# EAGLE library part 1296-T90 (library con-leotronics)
1.27mm SINGLE ROW FEMALE SOCKET Source: http://www.leotronics.co.uk/Conexcon/Data%20Sheets/sec.%20A/1296ing.pdf
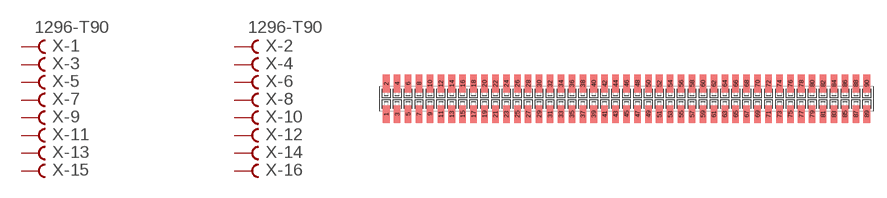
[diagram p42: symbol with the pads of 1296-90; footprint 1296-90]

Designator prefix X; gates -1=FVAL -2=FVAL -3=F -4=F -5=F -6=F -7=F -8=F -9=F -10=F -11=F -12=F -13=F -14=F -15=F -16=F -17=F -18=F -19=F -20=F -21=F -22=F -23=F -24=F -25=F -26=F -27=F -28=F -29=F -30=F -31=F -32=F -33=F -34=F -35=F -36=F -37=F -38=F -39=F -40=F -41=F -42=F -43=F -44=F -45=F -46=F -47=F -48=F -49=F -50=F -51=F -52=F -53=F -54=F -55=F -56=F -57=F -58=F -59=F -60=F -61=F -62=F -63=F -64=F -65=F -66=F -67=F -68=F -69=F -70=F -71=F -72=F -73=F -74=F -75=F -76=F -77=F -78=F -79=F -80=F -81=F -82=F -83=F -84=F -85=F -86=F -87=F -88=F -89=F -90=F

## 1296-T90 (OC_FARNELL: unknown; OC_NEWARK: unknown)  [1296-90]
1  -1:B  pas
2  -2:B  pas
3  -3:B  pas
4  -4:B  pas
5  -5:B  pas
6  -6:B  pas
7  -7:B  pas
8  -8:B  pas
9  -9:B  pas
10  -10:B  pas
11  -11:B  pas
12  -12:B  pas
13  -13:B  pas
14  -14:B  pas
15  -15:B  pas
16  -16:B  pas
17  -17:B  pas
18  -18:B  pas
19  -19:B  pas
20  -20:B  pas
21  -21:B  pas
22  -22:B  pas
23  -23:B  pas
24  -24:B  pas
25  -25:B  pas
26  -26:B  pas
27  -27:B  pas
28  -28:B  pas
29  -29:B  pas
30  -30:B  pas
31  -31:B  pas
32  -32:B  pas
33  -33:B  pas
34  -34:B  pas
35  -35:B  pas
36  -36:B  pas
37  -37:B  pas
38  -38:B  pas
39  -39:B  pas
40  -40:B  pas
41  -41:B  pas
42  -42:B  pas
43  -43:B  pas
44  -44:B  pas
45  -45:B  pas
46  -46:B  pas
47  -47:B  pas
48  -48:B  pas
49  -49:B  pas
50  -50:B  pas
51  -51:B  pas
52  -52:B  pas
53  -53:B  pas
54  -54:B  pas
55  -55:B  pas
56  -56:B  pas
57  -57:B  pas
58  -58:B  pas
59  -59:B  pas
60  -60:B  pas
61  -61:B  pas
62  -62:B  pas
63  -63:B  pas
64  -64:B  pas
65  -65:B  pas
66  -66:B  pas
67  -67:B  pas
68  -68:B  pas
69  -69:B  pas
70  -70:B  pas
71  -71:B  pas
72  -72:B  pas
73  -73:B  pas
74  -74:B  pas
75  -75:B  pas
76  -76:B  pas
77  -77:B  pas
78  -78:B  pas
79  -79:B  pas
80  -80:B  pas
81  -81:B  pas
82  -82:B  pas
83  -83:B  pas
84  -84:B  pas
85  -85:B  pas
86  -86:B  pas
87  -87:B  pas
88  -88:B  pas
89  -89:B  pas
90  -90:B  pas

## Footprint 1296-90 (pad centres in mm)
1.27mm SINGLE ROW FEMALE SOCKET Source: http://www.leotronics.co.uk/Conexcon/Data%20Sheets/sec.%20A/1296ing.pdf
smd 0.76 x 2.05: 1 -27.94,-1.78; 2 -27.94,1.78; 3 -26.67,-1.78; 4 -26.67,1.78; 5 -25.4,-1.78; 6 -25.4,1.78; 7 -24.13,-1.78; 8 -24.13,1.78; 9 -22.86,-1.78; 10 -22.86,1.78; 11 -21.59,-1.78; 12 -21.59,1.78; 13 -20.32,-1.78; 14 -20.32,1.78; 15 -19.05,-1.78; 16 -19.05,1.78; 17 -17.78,-1.78; 18 -17.78,1.78; 19 -16.51,-1.78; 20 -16.51,1.78; 21 -15.24,-1.78; 22 -15.24,1.78; 23 -13.97,-1.78; 24 -13.97,1.78; 25 -12.7,-1.78; 26 -12.7,1.78; 27 -11.43,-1.78; 28 -11.43,1.78; 29 -10.16,-1.78; 30 -10.16,1.78; 31 -8.89,-1.78; 32 -8.89,1.78; 33 -7.62,-1.78; 34 -7.62,1.78; 35 -6.35,-1.78; 36 -6.35,1.78; 37 -5.08,-1.78; 38 -5.08,1.78; 39 -3.81,-1.78; 40 -3.81,1.78; 41 -2.54,-1.78; 42 -2.54,1.78; 43 -1.27,-1.78; 44 -1.27,1.78; 45 0,-1.78; 46 0,1.78; 47 1.27,-1.78; 48 1.27,1.78; 49 2.54,-1.78; 50 2.54,1.78; 51 3.81,-1.78; 52 3.81,1.78; 53 5.08,-1.78; 54 5.08,1.78; 55 6.35,-1.78; 56 6.35,1.78; 57 7.62,-1.78; 58 7.62,1.78; 59 8.89,-1.78; 60 8.89,1.78; 61 10.16,-1.78; 62 10.16,1.78; 63 11.43,-1.78; 64 11.43,1.78; 65 12.7,-1.78; 66 12.7,1.78; 67 13.97,-1.78; 68 13.97,1.78; 69 15.24,-1.78; 70 15.24,1.78; 71 16.51,-1.78; 72 16.51,1.78; 73 17.78,-1.78; 74 17.78,1.78; 75 19.05,-1.78; 76 19.05,1.78; 77 20.32,-1.78; 78 20.32,1.78; 79 21.59,-1.78; 80 21.59,1.78; 81 22.86,-1.78; 82 22.86,1.78; 83 24.13,-1.78; 84 24.13,1.78; 85 25.4,-1.78; 86 25.4,1.78; 87 26.67,-1.78; 88 26.67,1.78; 89 27.94,-1.78; 90 27.94,1.78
